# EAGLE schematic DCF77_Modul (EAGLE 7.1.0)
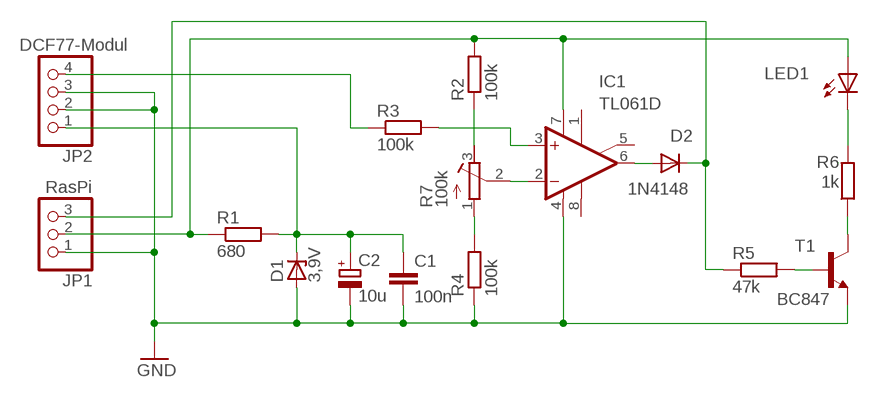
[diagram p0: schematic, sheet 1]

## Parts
C1  100n  C-EUC1206  [C1206]
C2  10u  CPOL-EUE1.8-4  [E1,8-4]
D1  3,9V  ZENER-DIODESOD80C  [SOD80C]
D2  1N4148  CGRM4001-G  [SOD-123_MINI-SMA]
IC1  TL061D  [SO08]
JP1  RasPi  PINHD-1X3  [1X03]
JP2  DCF77-Modul  PINHD-1X4  [1X04]
LED1  LEDCHIPLED_1206  [CHIPLED_1206]
R1  680  R-EU_M1206  [M1206]
R2  100k  R-EU_M1206  [M1206]
R3  100k  R-EU_M1206  [M1206]
R4  100k  R-EU_M1206  [M1206]
R5  47k  R-EU_M1206  [M1206]
R6  1k  R-EU_M1206  [M1206]
R7  100k  R-TRIMM4G/J  [RTRIM4G/J]
T1  BC847  [SOT23]

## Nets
3.9V: C1.1 C2.+ D1.C JP2.1 R1.2
DIGITALOUT: D2.C JP1.3 R5.1
GND: C1.2 C2.- D1.A IC1.4(V-) JP1.1 JP2.2 JP2.3 R4.1 T1.2(E)
N$1: JP2.4 R3.1
N$5: R4.2 R7.1(A)
N$6: R2.1 R7.3(E)
N$7: IC1.2(-IN) R7.2(S)
N$8: IC1.3(+IN) R3.2
N$11: D2.A IC1.6(OUT)
N$12: R5.2 T1.1(B)
N$13: R6.1 T1.3(C)
N$14: LED1.C R6.2
VCC: IC1.7(V+) JP1.2 LED1.A R1.1 R2.2
Unconnected: IC1.1(ON1) IC1.5(ON2) IC1.8(OPT)

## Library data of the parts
C1 = rcl:C-EU: CAPACITOR, European symbol
C2 = rcl:CPOL-EU: POLARIZED CAPACITOR, European symbol
D1 = diode:ZENER-DIODE: Z-Diode
D2 = diode:CGRM400*-G: Molded plasitc,JEDEC SOD-123/Mini SMA
IC1 = linear:TL061: OP AMP
JP1 = pinhead:PINHD-1X3: PIN HEADER
JP2 = pinhead:PINHD-1X4: PIN HEADER
LED1 = led:LED: LED
R1-R6 = rcl:R-EU_: RESISTOR, European symbol
R7 = rcl:R-TRIMM: Trimm resistor
T1 = transistor:BC847: NPN TRANSISTOR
